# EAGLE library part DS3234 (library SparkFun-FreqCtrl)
SPI RTC module with battery backup and internal clock.
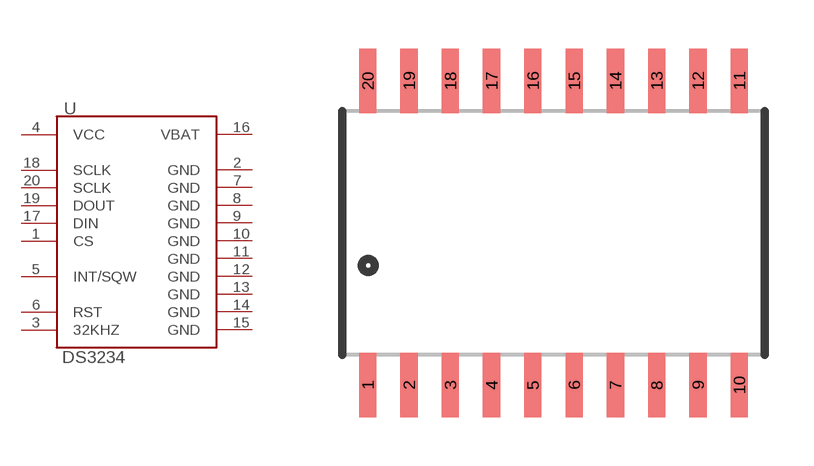
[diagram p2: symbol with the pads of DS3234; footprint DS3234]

Designator prefix -

## DS3234  [DS3234]
1  CS
2  GND
3  32KHZ
4  VCC
5  INT/SQW
6  RST
7  GND
8  GND
9  GND
10  GND
11  GND
12  GND
13  GND
14  GND
15  GND
16  VBAT
17  DIN
18  SCLK
19  DOUT
20  SCLK

## Footprint DS3234 (pad centres in mm)
smd 0.53 x 1.98: 1 -5.715,-4.685; 2 -4.445,-4.685; 3 -3.175,-4.685; 4 -1.905,-4.685; 5 -0.635,-4.685; 6 0.635,-4.685; 7 1.905,-4.685; 8 3.175,-4.685; 9 4.445,-4.685; 10 5.715,-4.685; 11 5.715,4.685; 12 4.445,4.685; 13 3.175,4.685; 14 1.905,4.685; 15 0.635,4.685; 16 -0.635,4.685; 17 -1.905,4.685; 18 -3.175,4.685; 19 -4.445,4.685; 20 -5.715,4.685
